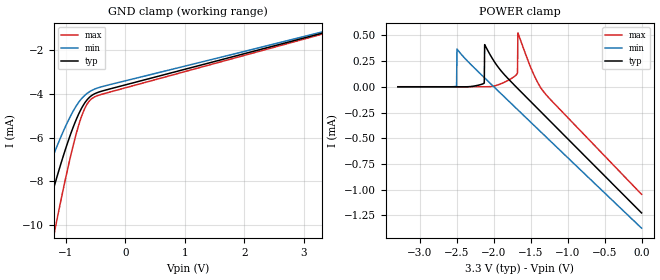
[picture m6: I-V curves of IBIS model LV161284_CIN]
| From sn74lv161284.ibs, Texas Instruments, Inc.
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[Model]   LV161284_CIN
Model_type  Input
Vinl=0.8
Vinh=2.3
| variable   typ   min   max
C_comp   1.66pF   1.31pF   1.95pF
[Temperature Range]   40   100   -40
| Ambient temperature   25   85   -40
[Voltage range]   3.3   3   3.6
[GND Clamp]
| LV161284_CIN
|   Voltage   I(typ)   I(min)   I(max)
-3.3V     -34.87mA   -25.82mA   -43.84mA
-1.665V   -13.26mA   -10.32mA   -17.32mA
-1.62V    -12.74mA   -9.952mA   -16.63mA
-1.415V   -10.48mA   -8.332mA   -13.56mA
-1.375V   -10.06mA   -8.029mA   -12.98mA
-1.18V    -8.111mA   -6.625mA   -10.21mA
-960mV    -6.172mA   -5.237mA   -7.348mA
-805mV    -5.059mA   -4.477mA   -5.643mA
-685mV    -4.434mA   -4.08mA    -4.695mA
-560mV    -4.068mA   -3.84mA    -4.215mA
-265mV    -3.779mA   -3.581mA   -3.922mA
3.3V      -1.226mA   -1.168mA   -1.269mA
[POWER Clamp]
| LV161284_CIN
|   Voltage   I(typ)   I(min)   I(max)
-3.3V     65.72nA    2.882nA    899.9nA
-2.505V   42.52nA    4.986uA    547.3nA
-2.5V     42.6nA     367uA      545.4nA
-2.13V    36.15uA    89.82uA    459.3nA
-2.125V   409.9uA    86.36uA    468.2nA
-1.94V    189.4uA    -41.39uA   20.28uA
-1.685V   -10.66uA   -217.2uA   127.6uA
-1.68V    -14.29uA   -220.7uA   136.1uA
-1.675V   -17.92uA   -224.1uA   524uA
-1.475V   -162.4uA   -361.8uA   144.1uA
-1.33V    -267.1uA   -461.6uA   -44.34uA
-48.03fV  -1.226mA   -1.373mA   -1.045mA
